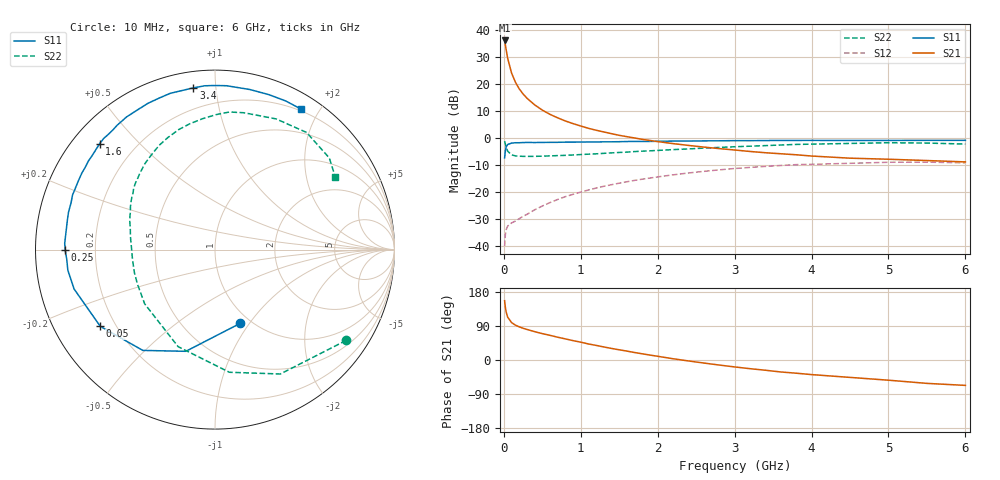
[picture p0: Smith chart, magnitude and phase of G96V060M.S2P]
! SIEMENS Small Signal Semiconductors
! BFG235
! Si NPN RF Bipolar Junction Transistor in SOT223
! VCE = 6 V  IC = 60 mA
! Common Emitter S-Parameters:  July  1994
# GHz  S  MA  R  50
!  f  S11  S21  S12  S22
! GHz  MAG  ANG  MAG  ANG  MAG  ANG  MAG  ANG
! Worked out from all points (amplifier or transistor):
!   40 points, 10 MHz to 6 GHz, reference 50 ohm
!   highest |S21| = 36.2 dB at 10 MHz (marker M1)
!   |S21| within 3 dB of that: start of sweep to 27.63 MHz
!   unconditionally stable (mu >= 1): 498.2 MHz to 1.402 GHz
!   at 200 MHz: K = 0.71, MSG = 24.0 dB, |S12| = -29.7 dB
!   at 1.5 GHz: K = 0.99, MSG = 8.9 dB, |S12| = -16.6 dB
!   at 6 GHz: K = 0.91, MSG = 0.2 dB, |S12| = -9.1 dB
!   S11 on the Smith chart (normalised r, x): 10 MHz: 0.90, -0.91; 50 MHz: 0.14, -0.30; 250 MHz: 0.09, -0.00; 1.6 GHz: 0.08, +0.39; 3.4 GHz: 0.08, +0.87; 6 GHz: 0.18, +1.77
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0.01  0.434 -70.9  64.66 156.5  0.0101 67.7  0.8888 -34.7
0.02  0.5895 -106.0  53.4 138.9  0.0166 53.2  0.7828 -62.3
0.03  0.6908 -125.6  43.63 126.8  0.0203 43.4  0.6881 -83.3
0.05  0.7689 -146.2  30.1 112.9  0.0238 34.2  0.5784 -110.8
0.1  0.8152 -164.4  16.23 98.9  0.0272 32.1  0.4949 -142.3
0.15  0.8279 -172.0  10.96 92.0  0.0294 35.8  0.473 -156.0
0.2  0.8279 -176.4  8.219 87.5  0.0326 39.6  0.4671 -163.8
0.25  0.8346 -179.8  6.624 83.7  0.0361 42.7  0.4635 -168.9
0.3  0.8381 177.6  5.533 80.7  0.0391 46.1  0.463 -173.0
0.4  0.8359 172.7  4.164 74.8  0.0475 50.3  0.4637 -178.6
0.5  0.8386 168.8  3.327 69.6  0.0559 52.8  0.4672 177.1
0.6  0.8423 165.7  2.774 65.1  0.0647 53.9  0.473 173.3
0.7  0.8432 162.0  2.391 60.1  0.0739 54.4  0.4786 170.1
0.9  0.8498 156.5  1.87 51.1  0.0921 53.1  0.4918 164.2
1.1  0.8557 150.0  1.53 42.3  0.1106 51.1  0.509 158.6
1.6  0.8723 137.4  1.072 23.5  0.1571 42.6  0.5556 145.2
2.2  0.8883 123.7  0.798 3.3  0.2108 30.3  0.6183 129.1
3.2  0.9049 101.9  0.571 -22.9  0.2895 6.8  0.7148 101.4
3.4  0.9092 97.6  0.541 -27.0  0.3021 1.9  0.7325 95.4
4.5  0.9127 77.7  0.429 -45.9  0.3448 -24.0  0.8037 65.0
5.5  0.9171 64.5  0.388 -61.7  0.3626 -46.5  0.8163 38.7
6  0.918 58.5  0.366 -67.0  0.3515 -54.8  0.783 31.2
